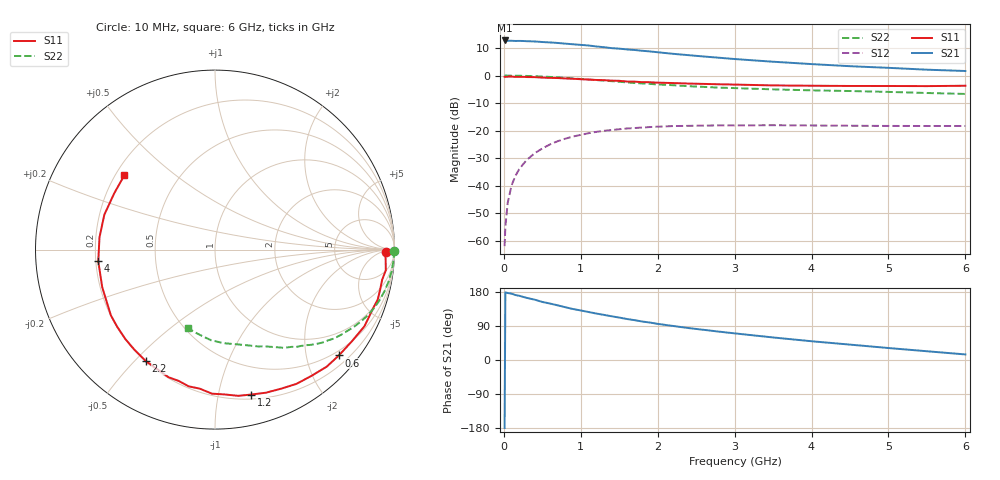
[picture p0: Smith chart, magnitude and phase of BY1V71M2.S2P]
! SIEMENS Small Signal Semiconductors
! BFY420
! Si NPN RF SIEGET Grounded Emitter Transistor in MICRO-X
! VCE = 1.75 V  IC = 1.2 mA
! Common Emitter S-Parameters:  October  1996
# GHz  S  MA  R  50
!  f  S11  S21  S12  S22
! GHz  MAG  ANG  MAG  ANG  MAG  ANG  MAG  ANG
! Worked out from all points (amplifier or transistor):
!   36 points, 10 MHz to 6 GHz, reference 50 ohm
!   highest |S21| = 12.7 dB at 10 MHz (marker M1)
!   |S21| within 3 dB of that: start of sweep to 1.51 GHz
!   unconditionally stable (mu >= 1): 4.416 GHz to end of sweep
!   at 250 MHz: K = 0.04, MSG = 22.4 dB, |S12| = -32.2 dB
!   at 1.4 GHz: K = 0.23, MSG = 14.9 dB, |S12| = -19.8 dB
!   at 6 GHz: K = 1.31, MAG = 6.6 dB, |S12| = -18.3 dB
!   S11 on the Smith chart (normalised r, x): 10 MHz: 37, -10; 600 MHz: 0.40, -2.66; 1.2 GHz: 0.24, -1.25; 2.2 GHz: 0.20, -0.54; 4 GHz: 0.21, -0.05; 6 GHz: 0.24, +0.34
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0.01  0.9515 -0.8  4.337 -179.4  0.0008 94.7  0.9999 -0.3
0.02  0.9491 -1.4  4.305 178.7  0.0018 87.3  0.9999 -0.7
0.05  0.9526 -3.5  4.274 176.8  0.0049 87.2  0.9971 -1.7
0.1  0.9587 -6.9  4.279 175.1  0.0101 87.6  0.9963 -3.5
0.15  0.9464 -10.2  4.246 171.4  0.0151 81.6  0.9935 -5.2
0.25  0.9484 -17.0  4.242 166.6  0.0245 79.5  0.9869 -8.6
0.4  0.9359 -27.1  4.159 159.3  0.0389 73.5  0.9729 -13.7
0.5  0.918 -33.8  4.062 153.2  0.0474 69.5  0.9599 -17.0
0.6  0.9079 -40.5  3.993 149.0  0.0563 65.6  0.944 -20.2
0.9  0.8751 -58.7  3.696 134.5  0.0783 54.5  0.8867 -28.9
1.1  0.8463 -70.4  3.515 126.7  0.0898 48.3  0.8473 -34.1
1.2  0.8325 -75.9  3.38 122.7  0.0949 45.2  0.8282 -36.7
1.4  0.8087 -86.2  3.148 115.4  0.1027 39.6  0.7912 -40.9
1.8  0.7591 -105.5  2.817 101.5  0.1139 30.3  0.7191 -48.3
2.2  0.7313 -121.7  2.482 89.8  0.1211 22.5  0.6682 -55.0
2.4  0.7161 -128.8  2.345 84.3  0.1223 19.7  0.641 -58.0
2.8  0.6941 -141.7  2.106 74.8  0.1246 14.3  0.6033 -63.2
3.5  0.6624 -161.5  1.783 59.5  0.1256 7.7  0.5617 -71.6
4  0.6536 -174.3  1.616 49.5  0.1242 4.4  0.5389 -77.9
4.5  0.6472 173.9  1.479 40.6  0.1228 1.7  0.5238 -84.6
5.5  0.6432 150.7  1.278 23.1  0.1215 -0.5  0.4823 -100.2
6  0.6535 140.5  1.21 14.7  0.1216 -0.2  0.4638 -109.2
